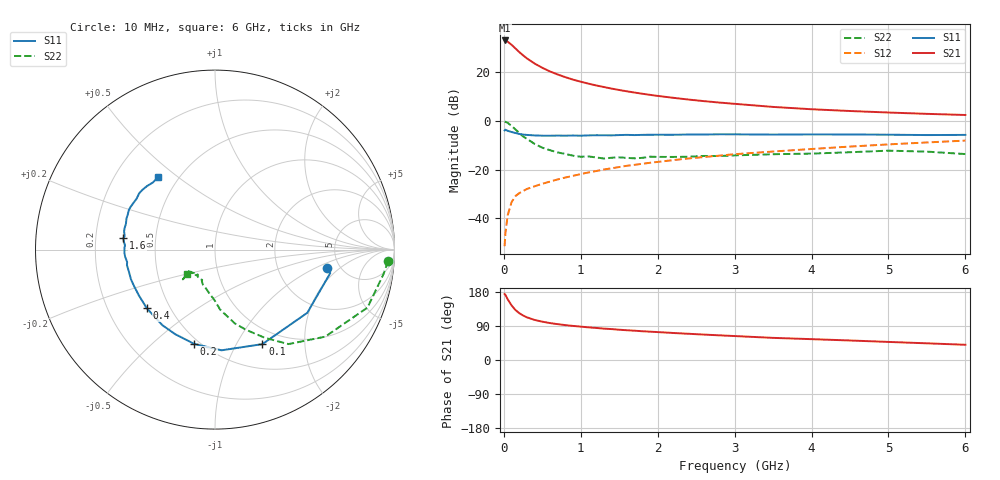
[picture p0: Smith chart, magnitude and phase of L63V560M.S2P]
!  INFINEON TECHNOLOGIES Small Signal Semiconductors
! BFR380L3 , Si-NPN RF-Transistor in TSLP-3-1
!  Vce=3.5 V,  Ic=60 mA
! Common Emitter S-Parameters:  07. March 2005
#  GHz  S  MA  R  50
! f  S11  S21  S12  S22
! GHz  Mag  Ang  Mag  Ang  Mag  Ang  Mag  Ang
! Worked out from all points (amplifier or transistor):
!   36 points, 10 MHz to 6 GHz, reference 50 ohm
!   highest |S21| = 32.9 dB at 10 MHz (marker M1)
!   |S21| within 3 dB of that: start of sweep to 141.6 MHz
!   unconditionally stable (mu >= 1): 1.52 GHz to 4.798 GHz
!   at 250 MHz: K = 0.50, MSG = 27.8 dB, |S12| = -28.8 dB
!   at 1.4 GHz: K = 1.00, MSG = 16.3 dB, |S12| = -19.5 dB
!   at 6 GHz: K = 0.97, MSG = 5.2 dB, |S12| = -8.1 dB
!   S11 on the Smith chart (normalised r, x): 10 MHz: 3.95, -1.38; 100 MHz: 0.80, -1.29; 200 MHz: 0.47, -0.69; 400 MHz: 0.37, -0.33; 1.6 GHz: 0.32, +0.05; 6 GHz: 0.39, +0.43
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0.01  0.6334 -9.5  44.17 174.1  0.0027 83.2  0.9663 -3.8
0.02  0.6554 -11.5  44.02 172.1  0.0049 86.6  0.9486 -8.3
0.05  0.6233 -34.4  41.67 160.2  0.0116 76.0  0.9091 -20.8
0.1  0.589 -63.4  36.08 144.2  0.0214 65.4  0.7826 -38.3
0.15  0.5623 -86.3  30.38 132.1  0.0286 59.3  0.6671 -52.1
0.2  0.5378 -102.5  25.59 123.6  0.0329 57.4  0.5651 -60.5
0.25  0.521 -115.1  21.93 117.5  0.0363 54.4  0.4786 -68.9
0.3  0.5132 -124.9  18.95 112.6  0.0401 54.9  0.4266 -74.9
0.4  0.5013 -139.3  14.87 105.7  0.0455 55.5  0.3356 -85.1
0.5  0.495 -148.8  12.17 101.1  0.0512 57.1  0.2811 -90.6
0.6  0.4947 -155.6  10.23 97.4  0.0568 59.1  0.2495 -96.6
0.7  0.4968 -160.7  8.872 94.6  0.0629 60.8  0.2245 -102.4
0.9  0.4982 -170.0  6.957 89.9  0.0746 63.0  0.1923 -112.3
1.1  0.502 -175.3  5.756 86.1  0.0875 64.5  0.1859 -117.7
1.3  0.5046 179.1  4.913 82.8  0.1004 65.6  0.1686 -125.2
1.6  0.5144 173.0  4.01 78.5  0.1196 66.4  0.1737 -132.6
2.2  0.5168 163.7  2.957 71.3  0.1563 66.9  0.1816 -134.5
2.8  0.528 155.2  2.363 65.1  0.193 66.6  0.1894 -140.6
3.5  0.5209 146.7  1.922 58.4  0.2344 64.4  0.2066 -138.9
4.5  0.524 140.7  1.585 51.5  0.2964 62.6  0.2268 -137.9
5.5  0.5096 132.9  1.386 44.0  0.36 58.7  0.2333 -137.4
6  0.5137 127.8  1.313 40.2  0.3928 56.5  0.2081 -139.4
